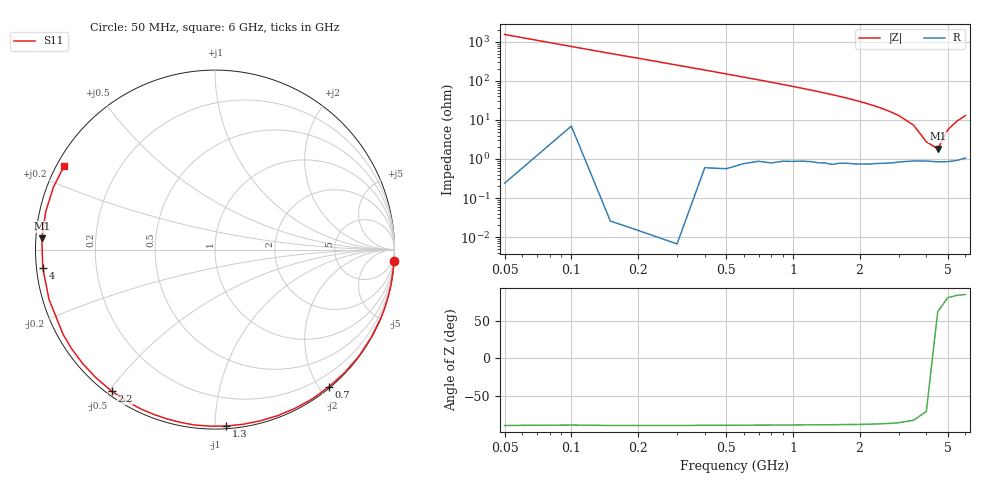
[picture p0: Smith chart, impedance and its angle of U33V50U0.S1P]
! SIEMENS Discrete & RF Semiconductors
! BBY53-02W
! Si Tuning Diode in SCD-80
! VR = 3.5 V
! S-Parameters:  September  1997
# GHz  S  MA  R  50
!  f  S11
! GHz  MAG  ANG
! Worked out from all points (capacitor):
!   34 points, 50 MHz to 6 GHz, reference 50 ohm
!   read as one part to ground: C = 2.09 pF near 50 MHz
!   lowest |Z| = 1.82 ohm at 4.5 GHz (marker M1)
!   series resonance near 4.309 GHz, so ESL is about 650 pH
!   S11 on the Smith chart (normalised r, x): 50 MHz: 0, -31; 700 MHz: 0.02, -2.13; 1.3 GHz: 0.02, -1.06; 2.2 GHz: 0.01, -0.51; 4 GHz: 0.02, -0.05; 6 GHz: 0.02, +0.26
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0.05  1 -3.7
0.2  1 -14.9
0.3  1 -22.3
0.4  0.9984 -29.5
0.5  0.9978 -36.6
0.6  0.9958 -43.6
0.7  0.9937 -50.3
0.8  0.9928 -56.9
0.9  0.9904 -63.3
1  0.9888 -69.3
1.1  0.9869 -75.2
1.2  0.9857 -80.9
1.3  0.9851 -86.4
1.5  0.984 -96.6
1.6  0.9817 -101.3
1.7  0.9802 -105.8
1.9  0.9791 -114.5
2.2  0.9767 -126.1
2.4  0.9744 -133.0
2.6  0.973 -139.4
2.8  0.9713 -145.4
3  0.9691 -150.9
3.5  0.9657 -163.3
4  0.9651 -174.0
4.5  0.9667 176.3
5  0.9667 167.3
5.5  0.965 158.9
6  0.9611 151.0
